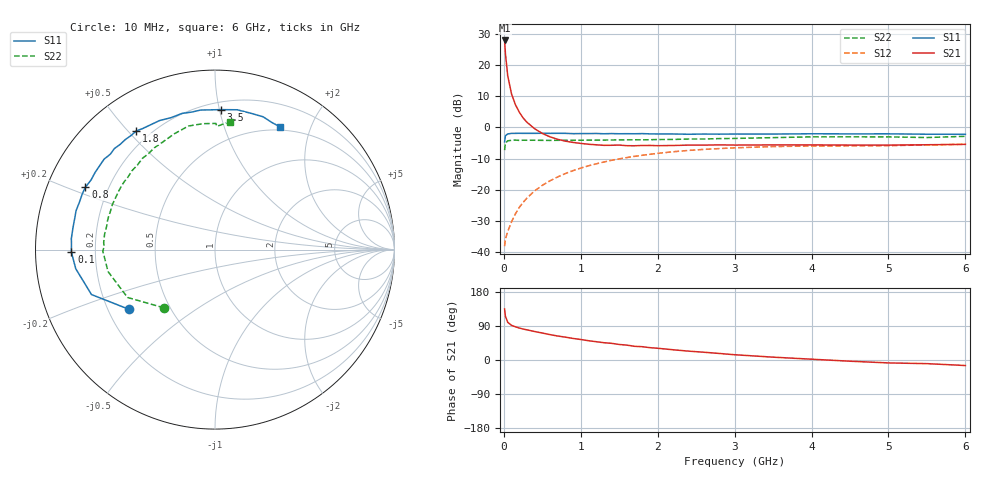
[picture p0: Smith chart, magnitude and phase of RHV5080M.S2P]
! SIEMENS Small Signal Semiconductors
! BFR106
! Si NPN RF Bipolar Junction Transistor in SOT23
! VCE = 0.5 V  IC = 80 mA
! Common Emitter S-Parameters:  August  1996
# GHz  S  MA  R  50
!  f  S11  S21  S12  S22
! GHz  MAG  ANG  MAG  ANG  MAG  ANG  MAG  ANG
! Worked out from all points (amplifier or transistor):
!   36 points, 10 MHz to 6 GHz, reference 50 ohm
!   highest |S21| = 27.8 dB at 10 MHz (marker M1)
!   |S21| within 3 dB of that: start of sweep to 17.48 MHz
!   unconditionally stable (mu >= 1): start of sweep to 13.16 MHz; 33.93 MHz to end of sweep
!   at 250 MHz: K = 1.75, MAG = 8.5 dB, |S12| = -24.1 dB
!   at 1.4 GHz: K = 1.30, MAG = -0.9 dB, |S12| = -10.6 dB
!   at 6 GHz: K = 1.04, MAG = -1.2 dB, |S12| = -5.4 dB
!   S11 on the Smith chart (normalised r, x): 10 MHz: 0.29, -0.29; 100 MHz: 0.11, -0.01; 800 MHz: 0.12, +0.23; 1.8 GHz: 0.15, +0.53; 3.5 GHz: 0.25, +1.01; 6 GHz: 0.46, +1.56
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0.01  0.5846 -145.4  24.61 134.6  0.0125 45.9  0.4314 -131.2
0.02  0.7323 -160.0  15.51 115.7  0.0162 38.4  0.5554 -151.3
0.05  0.7832 -172.2  6.746 99.6  0.0213 43.3  0.6084 -168.4
0.1  0.8003 -179.0  3.421 91.5  0.0307 53.7  0.6185 -176.5
0.15  0.8003 177.8  2.313 87.6  0.041 61.2  0.6253 -179.2
0.2  0.8027 175.6  1.757 84.4  0.0521 64.9  0.6178 178.4
0.25  0.8008 172.9  1.417 81.7  0.0626 66.8  0.6215 176.4
0.3  0.8007 171.4  1.207 79.6  0.0736 67.9  0.6208 175.1
0.4  0.8008 167.2  0.95 75.2  0.096 68.1  0.6212 172.3
0.5  0.8039 164.4  0.799 71.2  0.1177 67.6  0.6189 169.8
0.6  0.8002 160.7  0.704 67.0  0.1394 66.4  0.6174 167.6
0.8  0.8014 154.3  0.601 60.3  0.1817 63.0  0.6207 162.9
1.1  0.7947 144.0  0.536 50.9  0.242 57.0  0.6244 156.3
1.4  0.7944 134.9  0.516 44.0  0.2965 50.3  0.6274 149.5
1.8  0.7936 123.6  0.512 35.1  0.3571 41.8  0.6302 140.9
2.2  0.7825 113.3  0.512 27.0  0.4064 33.7  0.6395 132.4
2.6  0.7807 103.6  0.519 20.5  0.4431 26.1  0.6504 124.6
3.5  0.7805 87.6  0.523 7.5  0.4919 11.5  0.6839 109.4
4.5  0.7855 75.3  0.52 -3.2  0.5052 -1.1  0.7047 95.5
5  0.787 70.1  0.519 -7.7  0.5083 -5.9  0.703 89.6
5.5  0.7755 65.7  0.526 -9.6  0.5227 -8.2  0.6865 89.1
6  0.7743 62.1  0.534 -14.6  0.5349 -13.9  0.7181 83.5
